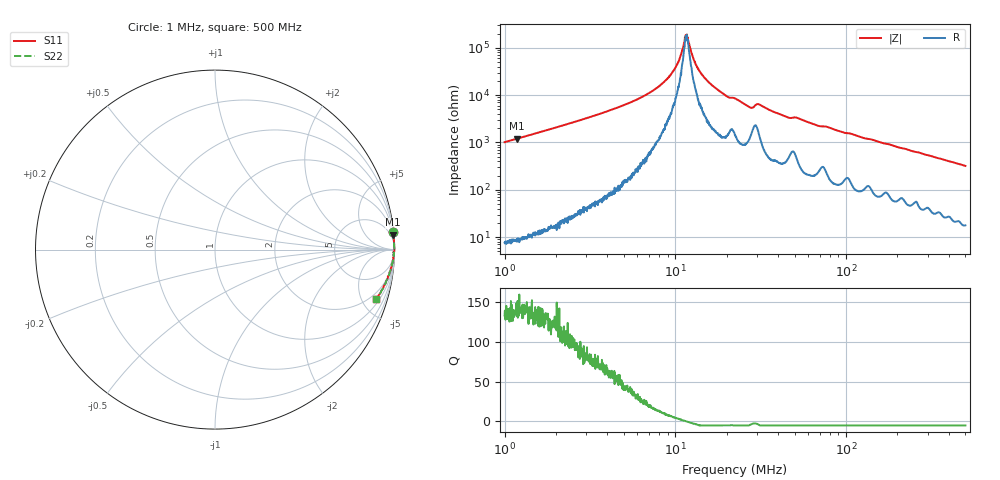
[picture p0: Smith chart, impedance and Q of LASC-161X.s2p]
!s-Parameter Generated by FASTRON Sdn. Bhd.
!FASTRON P/N : LASC-161X
!Keysight Technologies,E4991B,MY54100416,A.01.15
!Date: Tue Mar 17 15:23:48 2026
!Version  : Rev00 Tue Mar 17 15:23:48 2026
!Data & Calibration Information:
!PortZ  Port1:50+j0  Port2:50+j0
!When reading, reference impedance value at option line is always used.
! Remarks : This data is being provided solely for informational purposes.
!Freq	S11	S21	S12	S22
# Hz S dB R 50
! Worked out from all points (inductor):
!   1601 points, 1 MHz to 500 MHz, reference 50 ohm
!   read as one part in series: L = 160 uH near 1.032 MHz
!   highest Q = 140 at 1.182 MHz (marker M1), where L = 162 uH
!   self-resonance near 11.6 MHz
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1000000  -0.05 5.6  -20.18 -83.9  -20.18 -83.9  -0.05 5.6
1181775  -0.04 4.7  -21.64 -84.8  -21.64 -84.8  -0.04 4.7
2820919  -0.01 1.9  -29.61 -87.4  -29.61 -87.4  -0.01 1.9
5417295  -0.00 0.8  -36.85 -87.7  -36.85 -87.7  -0.00 0.8
7957584  -0.00 0.4  -43.55 -85.4  -43.55 -85.4  -0.00 0.4
9081014  -0.01 0.2  -47.38 -82.1  -47.38 -82.1  -0.01 0.2
1.000704e7  -0.01 0.1  -51.63 -76.9  -51.63 -76.9  -0.01 0.1
1.056627e7  -0.00 0.1  -55.19 -71.3  -55.19 -71.3  -0.00 0.1
1.133144e7  -0.00 0.0  -62.69 -39.0  -62.69 -39.0  -0.00 0.0
1.159862e7  -0.01 0.0  -64.75 -2.6  -64.75 -2.6  -0.01 0.0
1.18721e7  -0.01 -0.0  -63.10 30.5  -63.10 30.5  -0.01 -0.0
1.313366e7  -0.01 -0.1  -53.16 72.6  -53.16 72.6  -0.01 -0.1
1.452928e7  -0.01 -0.2  -48.21 79.8  -48.21 79.8  -0.01 -0.2
1.929232e7  -0.01 -0.5  -40.33 82.3  -40.33 82.3  -0.01 -0.5
2.236068e7  -0.02 -0.7  -38.67 79.8  -38.67 79.8  -0.02 -0.7
2.736538e7  -0.04 -1.0  -34.87 75.7  -34.87 75.7  -0.04 -1.0
3.086698e7  -0.03 -0.9  -36.16 75.6  -36.16 75.6  -0.03 -0.9
4.499032e7  -0.03 -1.6  -30.76 81.4  -30.76 81.4  -0.03 -1.6
5.154174e7  -0.04 -1.7  -30.48 80.7  -30.48 80.7  -0.04 -1.7
6.307767e7  -0.03 -2.3  -28.04 83.3  -28.04 83.3  -0.03 -2.3
1.77937e8  -0.13 -6.1  -19.38 79.1  -19.38 79.1  -0.13 -6.1
5e8  -0.54 -17.1  -10.63 69.7  -10.63 69.7  -0.54 -17.1
